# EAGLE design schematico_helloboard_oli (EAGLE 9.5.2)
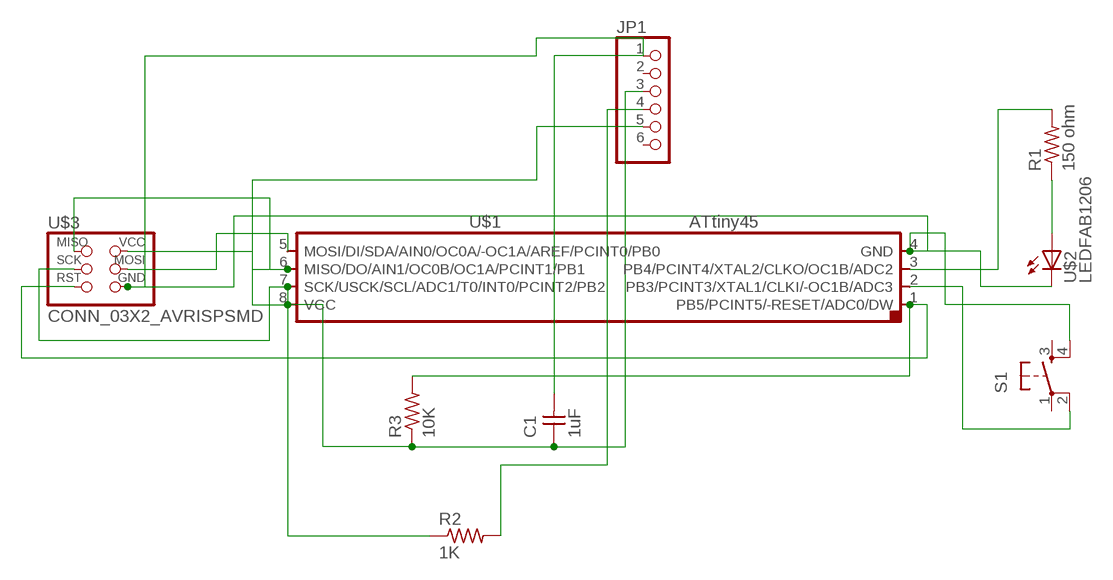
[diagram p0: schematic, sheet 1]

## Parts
C1  1uF  CAP_UNPOLARIZEDFAB  [C1206FAB]
JP1  PINHD-1X6  [1X06]
R1  150 ohm  R1206FAB  [R1206FAB]
R2  1K  R1206FAB  [R1206FAB]
R3  10K  R1206FAB  [R1206FAB]
S1  SW_SWITCH_TACTILE_6MM6MM_SWITCH  [6MM_SWITCH]
U$1  UC_ATTINY45SI  [SOIC8]
U$2  LEDFAB1206  [LED1206FAB]
U$3  CONN_03X2_AVRISPSMD  [2X03SMD]

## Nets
N$1: S1.2(P1) U$1.2(PB3/PCINT3/XTAL1/CLKI/-OC1B/ADC3)
N$2: R1.1 U$2.1(A)
N$3: R3.2 U$1.1(PB5/PCINT5/-RESET/ADC0/DW) U$3.5(RST)
N$4: C1.1 JP1.3 R2.1 R3.1 U$1.7(SCK/USCK/SCL/ADC1/T0/INT0/PCINT2/PB2) U$1.8(VCC) U$3.2(VCC) U$3.3(SCK)
N$5: U$1.5(MOSI/DI/SDA/AIN0/OC0A/-OC1A/AREF/PCINT0/PB0) U$3.4(MOSI)
N$6: R1.2 U$1.3(PB4/PCINT4/XTAL2/CLKO/OC1B/ADC2)
N$7: C1.2 JP1.1 S1.4(S1) U$1.4(GND) U$2.2(C) U$3.6(GND)
N$9: JP1.4 R2.2
N$11: JP1.5 U$1.6(MISO/DO/AIN1/OC0B/OC1A/PCINT1/PB1) U$3.1(MISO)
Unconnected: JP1.2 JP1.6 S1.1(P) S1.3(S)

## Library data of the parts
C1 = fab:CAP_UNPOLARIZED
JP1 = pinhead:PINHD-1X6: PIN HEADER
R1-R3 = fab:R: Resistor (US Symbol)
S1 = fab:SW_SWITCH_TACTILE_6MM: OMRON SWITCH
U$1 = fab:UC_ATTINY45
U$2 = fab:LED: LED
U$3 = fab:CONN_03X2_AVRISP

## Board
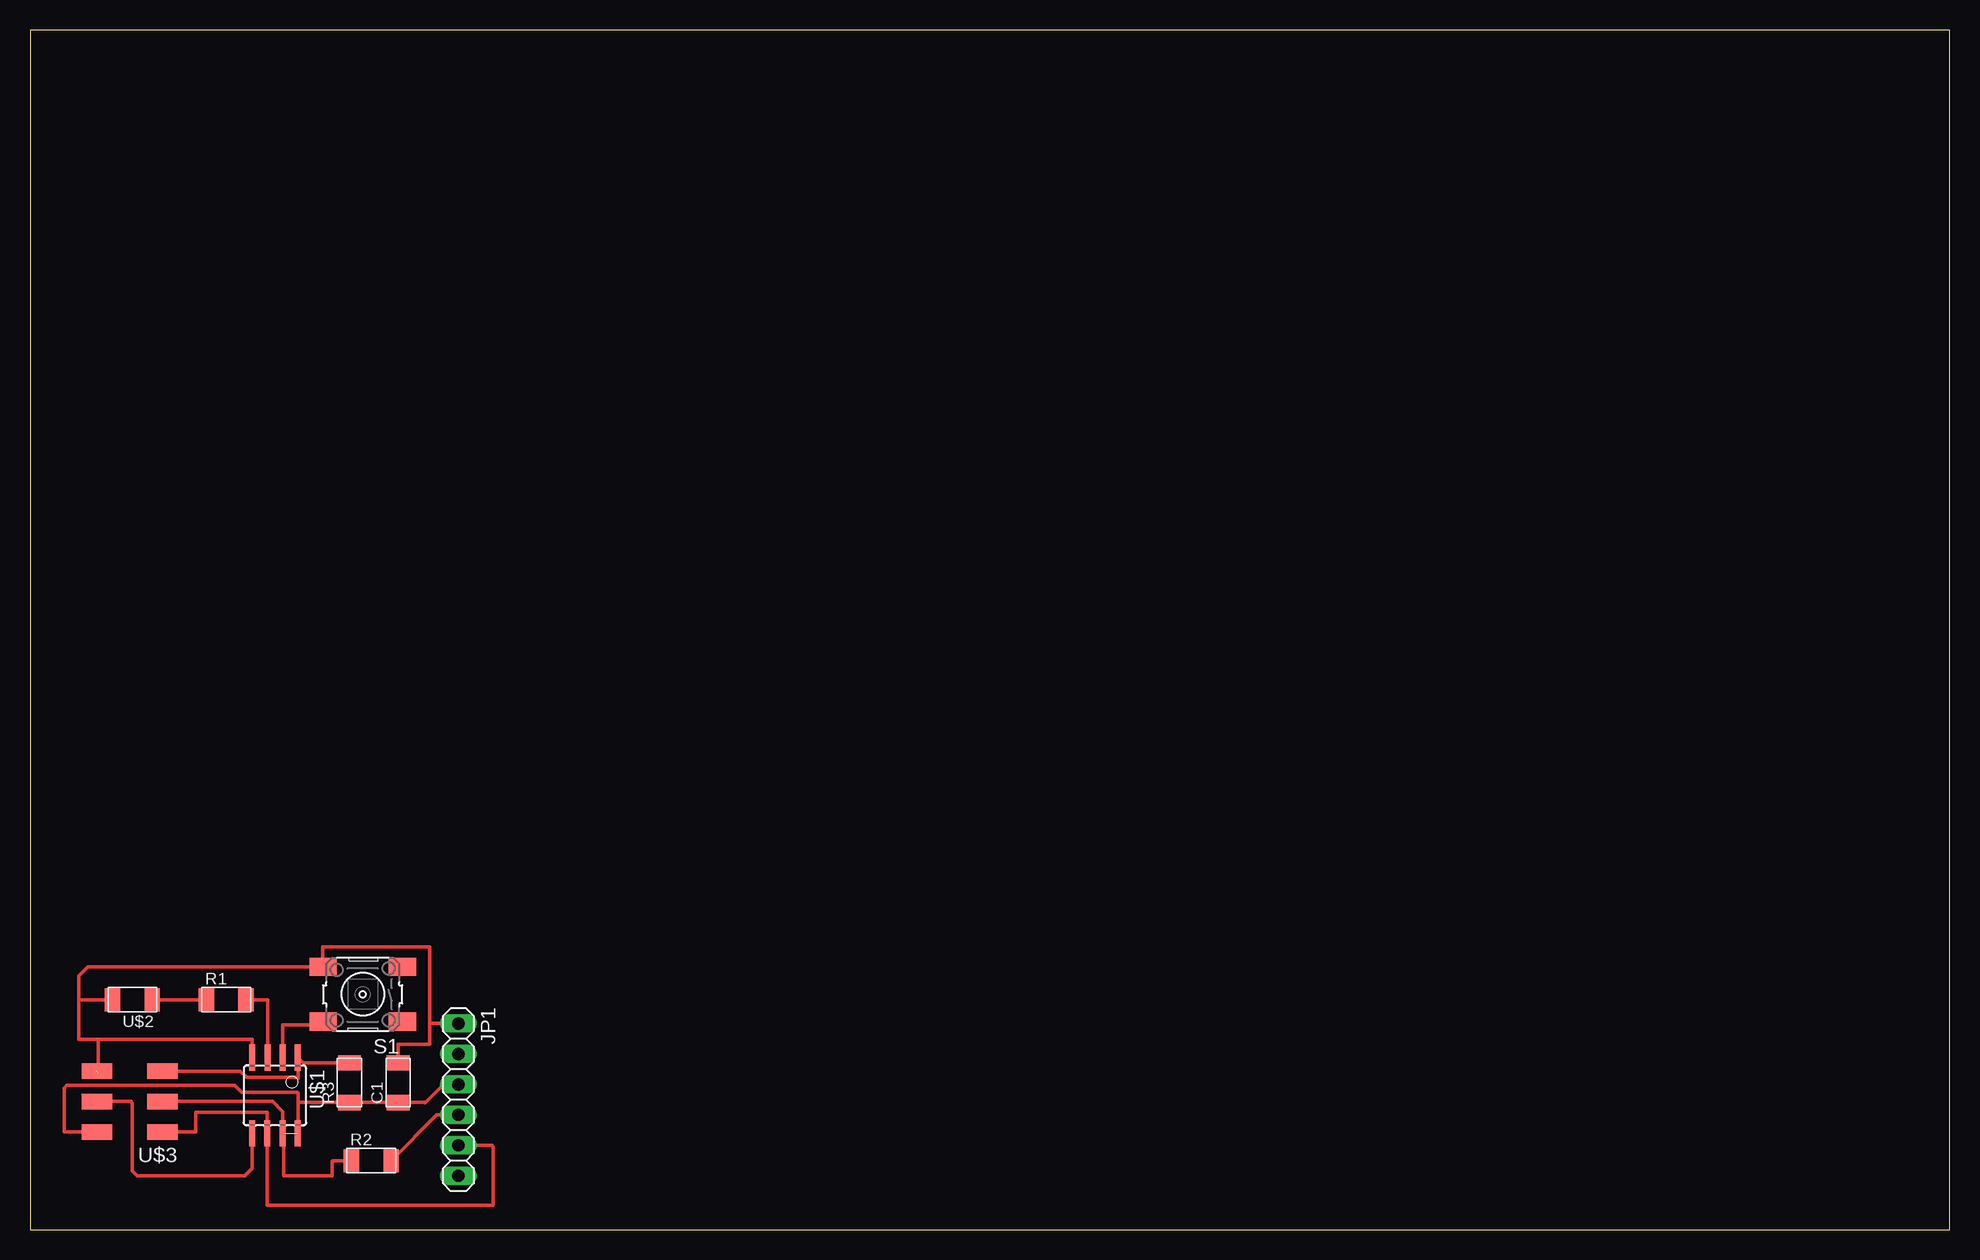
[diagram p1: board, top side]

Size 160 x 100 mm. Coordinates in mm from the lower left corner, seen from the top.
Outline: 0,0 160,0 160,100 0,100 0,0
Copper layers (1*16): Top 0.035mm / dielectric 0.15mm / Bottom 0.035mm
Design rules "default *": minimum track width 12mil, minimum drill 32mil, track to track 16mil, track to pad 16mil, pad to pad 16mil, via to via 16mil, smd to smd 16mil, copper to edge 16mil, drill to drill 16mil, minimum pad ring 10mil, minimum via ring 8mil, stop-mask expansion 4mil, vias tented up to drill 0mil, thermal gap 10mil

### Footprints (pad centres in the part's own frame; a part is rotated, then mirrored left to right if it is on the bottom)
C1206FAB = smd 1.27 x 1.905: 1 -1.651,0; 2 1.651,0
1X06 = drill 1.016 long: 1 -6.35,0; 2 -3.81,0; 3 -1.27,0; 4 1.27,0; 5 3.81,0; 6 6.35,0
R1206FAB = smd 1.27 x 1.905: 1 -1.651,0; 2 1.651,0
6MM_SWITCH = smd 2.286 x 1.524: 1 -3.302,2.286; 2 3.302,2.286; 3 -3.302,-2.286; 4 3.302,-2.286
SOIC8 = smd 0.5 x 2.2: 1 -1.905,-3.154; 2 -0.645,-3.154; 3 0.625,-3.154; 4 1.895,-3.154; 5 1.905,3.154; 6 0.635,3.154; 7 -0.635,3.154; 8 -1.905,3.154
LED1206FAB = smd 1.27 x 1.905: 1 -1.651,0; 2 1.651,0
2X03SMD = smd 2.54 x 1.27: 1 -2.54,2.54; 2 2.92,2.54; 3 -2.54,0; 4 2.92,0; 5 -2.54,-2.54; 6 2.92,-2.54

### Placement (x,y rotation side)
C1  30.68,12.24 90 top
JP1  35.71,10.82 270 top
R1  16.36,19.15 0 top
R2  28.45,5.74 0 top
R3  26.62,12.24 90 top
S1  27.74,19.61 180 top
U$1  20.42,11.18 180 top
U$2  8.53,19.15 180 top
U$3  8.48,10.67 180 top

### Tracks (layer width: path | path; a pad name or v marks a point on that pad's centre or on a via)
N$1
  Top 0.305: S1.2 24.43,17.07 21.07,17.07 U$1.2
N$2
  Top 0.305: R1.1 U$2.1
N$3
  Top 0.305: 26.59,13.92 R3.2 22.76,13.89 22.35,14.3 | U$3.5 17.51,13.21 18.05,12.67 22.28,12.67 22.35,12.6 22.35,14.3 | U$1.1 22.35,14.3
N$4  (1 unrouted)
  Top 0.305: JP1.3 35.61,12.19 34.54,12.19 32.92,10.57 32.89,10.59 C1.1 R3.1 22.35,10.59 | U$3.3 20.22,10.67 21.06,9.83 U$1.7 21.13,7.95 21.13,4.47 25.2,4.47 25.2,5.69 25.25,5.74 R2.1 | U$3.2 2.85,8.13 2.85,11.79 3.07,12.01 17.08,12.01 17.64,11.45 22.28,11.45 22.35,11.38 22.35,10.59 | 22.35,10.59 22.35,8.05 U$1.8
N$5
  Top 0.305: U$1.5 18.52,5.11 17.88,4.47 8.94,4.47 8.53,4.88 8.53,10.57 8.43,10.67 U$3.4
N$6
  Top 0.305: U$1.3 19.8,19.15 R1.2
N$7  (1 unrouted)
  Top 0.305: 5.69,15.85 18.53,15.85 U$1.4 | 5.69,13.01 5.69,15.85 | 4.06,19.15 4.06,21.13 4.83,21.89 S1.4 24.38,21.95 24.38,23.57 33.33,23.57 33.33,17.17 | 4.06,19.15 4.06,15.85 5.69,15.85 | C1.2 30.68,15.44 33.33,15.44 33.33,17.17 | JP1.1 33.33,17.17 | U$2.2 4.06,19.15
N$9
  Top 0.305: R2.2 33.91,9.55 JP1.4
N$11
  Top 0.305: JP1.5 38.51,7.01 38.61,6.91 38.61,2.03 19.79,2.03 U$1.6 19.79,9.75 13.82,9.75 13.82,8.13 U$3.1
